| TEXAS INSTRUMENTS INCORPORATED
| Standard Linear and Logic Group
| IBIS Model of SN74AHC04
| HEX INVERTERS
| This file contains package information for the following:
|  SOIC 14-pin (D) package as [Component] AHC04_D
|  SSOP 14-pin (DB) package as [Component] AHC04_DB
|  TVSOP 14-pin (DGV) package as [Component] AHC04_DGV
|  PDIP 14-pin (N) package as [Component] AHC04_N
|  SOP 14-pin (NS) package as [Component] AHC04_NS
|  TSSOP 14-pin (PW) package as [Component] AHC04_PW
|  QFN 14-pin (RGY) package as [Component] AHC04_RGY
| This device can be powered at the following Vccs:
|  3.3 volt Vcc
|  5 volt Vcc
| This file provides unique models under the [Model Selector] for each Vcc.
| For operation at a specific Vcc, select the appropriate model after each
| [Model Selector] keyword.
[IBIS Ver]   3.2
[Comment char]  |_char
[File Name]   sn74ahc04.ibs
[File Rev]   1.1 | b_die
[Date]   May 16, 2003
[Source]   Data created from TI-SPICE simulations at TI-SLL.
[Notes]   The following is an IBIS list for the AHC04.
   Please contact sllibis@ti.com with questions and
   comments concerning SLL IBIS models.
   This IBIS model is created from a BA (back annotated
   netlist).
   - Power-clamp data has been deleted from the input model
[Disclaimer] Property of Texas Instruments Incorporated.  Unauthorized
   reproduction and/or distribution is strictly prohibited.
   This product is protected under copyright law.
   Created  2003, (C) Copyright  2003, Texas Instruments
   Incorporated, All Rights Reserved
   UNLESS THERE IS A SIGNED, WRITTEN AGREEMENT TO THE
   CONTRARY, TEXAS INSTRUMENTS (TI) IS PROVIDING THE IBIS
   MODELS  AND WITHOUT ANY WARRANTY, EXPRESSED OR
   IMPLIED.  TI assumes no liability for:
   1) the accuracy of the IBIS models provided to your
   company;
   2) the proper functioning of these IBIS Models in your
   design or for any resulting applications; or
   3) infringement of patents, copyrights or intellectual
   property rights resulting from your use of these IBIS
   models.
   TI provides IBIS Models as a service to our customers.
   You and your company shall not distribute, sell or give
   these models to anyone else without prior written
   permission from TI.
   TI reserves the right to make changes to our products or
   to discontinue any semiconductor product or service
   without notice, and advises our customers to obtain the
   latest version of relevant information to verify, before
   placing orders, that the information being relied on is
   current.
   Please be aware that your receipt and use of the IBIS
   information provided shall serve as acceptance of these
   terms and conditions.  If you do not accept these terms,
   you should return or destroy the IBIS models and any
   other accompanying information immediately.
| Component AHC04_D 14-pin SOIC
[Component]   AHC04_D
[Manufacturer]   Texas Instruments, Inc.
[Package]
|   typ   min   max
R_pkg   3.100e-02   2.800e-02   3.400e-02
L_pkg   3.109e-09   2.462e-09   3.889e-09
C_pkg   4.730e-13   3.630e-13   6.280e-13
[Pin]   signal_name   model_name   R_pin   L_pin   C_pin
1   1A   AHC04_IN   3.300e-02   3.854e-09   6.220e-13
2   1Y   AHC04_OUT   3.200e-02   3.188e-09   4.730e-13
3   2A   AHC04_IN   2.800e-02   2.462e-09   3.770e-13
4   2Y   AHC04_OUT   3.100e-02   2.596e-09   3.630e-13
5   3A   AHC04_IN   2.800e-02   2.521e-09   3.720e-13
6   3Y   AHC04_OUT   3.400e-02   3.250e-09   4.760e-13
7   GND   GND   3.400e-02   3.889e-09   6.280e-13
8   4Y   AHC04_OUT   3.400e-02   3.889e-09   6.280e-13
9   4A   AHC04_IN   3.400e-02   3.250e-09   4.760e-13
10   5Y   AHC04_OUT   2.800e-02   2.521e-09   3.720e-13
11   5A   AHC04_IN   3.100e-02   2.596e-09   3.640e-13
12   6Y   AHC04_OUT   2.800e-02   2.462e-09   3.770e-13
13   6A   AHC04_IN   3.200e-02   3.188e-09   4.730e-13
14   VCC   POWER   3.300e-02   3.854e-09   6.220e-13
| Component AHC04_DB 14-pin SSOP
[Component]   AHC04_DB
[Manufacturer]   Texas Instruments, Inc.
[Package]
|   typ   min   max
R_pkg   4.400e-02   4.100e-02   4.600e-02
L_pkg   3.551e-09   3.258e-09   3.927e-09
C_pkg   4.020e-13   3.600e-13   4.210e-13
[Pin]   signal_name   model_name   R_pin   L_pin   C_pin
1   1A   AHC04_IN   4.600e-02   3.927e-09   4.080e-13
2   1Y   AHC04_OUT   4.400e-02   3.587e-09   4.210e-13
3   2A   AHC04_IN   4.100e-02   3.289e-09   3.980e-13
4   2Y   AHC04_OUT   4.200e-02   3.258e-09   3.600e-13
5   3A   AHC04_IN   4.100e-02   3.286e-09   4.030e-13
6   3Y   AHC04_OUT   4.400e-02   3.586e-09   4.210e-13
7   GND   GND   4.600e-02   3.927e-09   4.080e-13
8   4Y   AHC04_OUT   4.600e-02   3.927e-09   4.080e-13
9   4A   AHC04_IN   4.400e-02   3.586e-09   4.210e-13
10   5Y   AHC04_OUT   4.100e-02   3.286e-09   4.030e-13
11   5A   AHC04_IN   4.300e-02   3.258e-09   3.600e-13
12   6Y   AHC04_OUT   4.100e-02   3.289e-09   3.980e-13
13   6A   AHC04_IN   4.400e-02   3.587e-09   4.210e-13
14   VCC   POWER   4.600e-02   3.927e-09   4.080e-13
| Component AHC04_DGV 14-pin TVSOP
[Component]   AHC04_DGV
[Manufacturer]   Texas Instruments, Inc.
[Package]
|   typ   min   max
R_pkg   3.500e-02   2.000e-02   4.500e-02
L_pkg   2.499e-09   2.077e-09   2.966e-09
C_pkg   3.610e-13   3.050e-13   4.160e-13
[Pin]   signal_name   model_name   R_pin   L_pin   C_pin
1   1A   AHC04_IN   2.700e-02   2.717e-09   3.730e-13
2   1Y   AHC04_OUT   3.700e-02   2.434e-09   3.980e-13
3   2A   AHC04_IN   3.400e-02   2.200e-09   3.160e-13
4   2Y   AHC04_OUT   2.000e-02   2.077e-09   3.090e-13
5   3A   AHC04_IN   3.000e-02   2.147e-09   3.050e-13
6   3Y   AHC04_OUT   4.200e-02   2.580e-09   4.080e-13
7   GND   GND   3.900e-02   2.921e-09   3.850e-13
8   4Y   AHC04_OUT   3.300e-02   2.841e-09   3.800e-13
9   4A   AHC04_IN   4.200e-02   2.611e-09   4.100e-13
10   5Y   AHC04_OUT   3.800e-02   2.331e-09   3.290e-13
11   5A   AHC04_IN   2.600e-02   2.223e-09   3.190e-13
12   6Y   AHC04_OUT   3.400e-02   2.259e-09   3.130e-13
13   6A   AHC04_IN   4.500e-02   2.681e-09   4.160e-13
14   VCC   POWER   4.200e-02   2.966e-09   3.860e-13
| Component AHC04_N 14-pin PDIP
[Component]   AHC04_N
[Manufacturer]   Texas Instruments, Inc.
[Package]
|   typ   min   max
R_pkg   4.500e-02   3.700e-02   6.300e-02
L_pkg   5.407e-09   3.922e-09   6.942e-09
C_pkg   3.890e-13   2.050e-13   6.040e-13
[Pin]   signal_name   model_name   R_pin   L_pin   C_pin
1   1A   AHC04_IN   6.300e-02   6.942e-09   6.040e-13
2   1Y   AHC04_OUT   3.700e-02   6.200e-09   4.060e-13
3   2A   AHC04_IN   4.200e-02   4.389e-09   3.220e-13
4   2Y   AHC04_OUT   3.800e-02   3.922e-09   2.050e-13
5   3A   AHC04_IN   3.900e-02   4.301e-09   2.980e-13
6   3Y   AHC04_OUT   3.800e-02   5.329e-09   3.560e-13
7   GND   GND   5.300e-02   6.510e-09   5.440e-13
8   4Y   AHC04_OUT   5.300e-02   6.437e-09   5.390e-13
9   4A   AHC04_IN   3.900e-02   5.352e-09   3.470e-13
10   5Y   AHC04_OUT   4.200e-02   4.473e-09   2.970e-13
11   5A   AHC04_IN   4.400e-02   4.326e-09   2.250e-13
12   6Y   AHC04_OUT   4.200e-02   4.295e-09   2.800e-13
13   6A   AHC04_IN   4.200e-02   6.318e-09   4.180e-13
14   VCC   POWER   6.100e-02   6.900e-09   6.030e-13
| Component AHC04_NS 14-pin SOP
[Component]   AHC04_NS
[Manufacturer]   Texas Instruments, Inc.
[Package]
|   typ   min   max
R_pkg   4.500e-02   3.900e-02   5.400e-02
L_pkg   3.796e-09   2.561e-09   4.952e-09
C_pkg   5.280e-13   2.880e-13   7.100e-13
[Pin]   signal_name   model_name   R_pin   L_pin   C_pin
1   1A   AHC04_IN   4.700e-02   4.867e-09   7.060e-13
2   1Y   AHC04_OUT   5.100e-02   4.083e-09   5.920e-13
3   2A   AHC04_IN   4.100e-02   2.915e-09   3.760e-13
4   2Y   AHC04_OUT   3.900e-02   2.561e-09   2.880e-13
5   3A   AHC04_IN   4.100e-02   3.101e-09   4.300e-13
6   3Y   AHC04_OUT   4.700e-02   4.047e-09   5.890e-13
7   GND   GND   5.100e-02   4.909e-09   7.000e-13
8   4Y   AHC04_OUT   4.500e-02   4.784e-09   6.940e-13
9   4A   AHC04_IN   5.400e-02   4.176e-09   5.970e-13
10   5Y   AHC04_OUT   3.900e-02   3.287e-09   4.490e-13
11   5A   AHC04_IN   3.900e-02   2.586e-09   2.940e-13
12   6Y   AHC04_OUT   4.000e-02   2.802e-09   3.710e-13
13   6A   AHC04_IN   4.900e-02   4.080e-09   5.930e-13
14   VCC   POWER   5.200e-02   4.952e-09   7.100e-13
| Component AHC04_PW 14-pin TSSOP
[Component]   AHC04_PW
[Manufacturer]   Texas Instruments, Inc.
[Package]
|   typ   min   max
R_pkg   3.200e-02   2.900e-02   3.500e-02
L_pkg   2.378e-09   2.170e-09   2.680e-09
C_pkg   3.140e-13   2.700e-13   3.350e-13
[Pin]   signal_name   model_name   R_pin   L_pin   C_pin
1   1A   AHC04_IN   3.300e-02   2.618e-09   3.300e-13
2   1Y   AHC04_OUT   3.100e-02   2.313e-09   3.170e-13
3   2A   AHC04_IN   3.000e-02   2.310e-09   3.140e-13
4   2Y   AHC04_OUT   3.100e-02   2.173e-09   2.720e-13
5   3A   AHC04_IN   3.000e-02   2.204e-09   3.090e-13
6   3Y   AHC04_OUT   3.200e-02   2.315e-09   3.170e-13
7   GND   GND   3.500e-02   2.680e-09   3.350e-13
8   4Y   AHC04_OUT   3.300e-02   2.640e-09   3.330e-13
9   4A   AHC04_IN   3.400e-02   2.347e-09   3.190e-13
10   5Y   AHC04_OUT   2.900e-02   2.277e-09   3.130e-13
11   5A   AHC04_IN   3.100e-02   2.170e-09   2.700e-13
12   6Y   AHC04_OUT   3.100e-02   2.244e-09   3.110e-13
13   6A   AHC04_IN   3.300e-02   2.343e-09   3.210e-13
14   VCC   POWER   3.500e-02   2.657e-09   3.320e-13
| Component AHC04_RGY 14-pin QFN
[Component]   AHC04_RGY
[Manufacturer]   Texas Instruments, Inc.
[Package]
|   typ   min   max
R_pkg   2.900e-02   2.300e-02   4.100e-02
L_pkg   7.730e-10   6.570e-10   9.980e-10
C_pkg   1.360e-13   1.150e-13   1.560e-13
[Pin]   signal_name   model_name   R_pin   L_pin   C_pin
1   1A   AHC04_IN   2.700e-02   8.310e-10   1.300e-13
2   1Y   AHC04_OUT   2.700e-02   8.660e-10   1.350e-13
3   2A   AHC04_IN   4.100e-02   9.980e-10   1.560e-13
4   2Y   AHC04_OUT   3.100e-02   7.670e-10   1.420e-13
5   3A   AHC04_IN   3.100e-02   7.650e-10   1.420e-13
6   3Y   AHC04_OUT   3.100e-02   7.830e-10   1.440e-13
7   GND   GND   3.100e-02   7.810e-10   1.370e-13
8   4Y   AHC04_OUT   2.300e-02   6.570e-10   1.150e-13
9   4A   AHC04_IN   2.300e-02   8.140e-10   1.290e-13
10   5Y   AHC04_OUT   2.800e-02   7.040e-10   1.290e-13
11   5A   AHC04_IN   2.700e-02   6.720e-10   1.360e-13
12   6Y   AHC04_OUT   2.700e-02   6.960e-10   1.380e-13
13   6A   AHC04_IN   2.700e-02   7.250e-10   1.400e-13
14   VCC   POWER   3.000e-02   7.630e-10   1.360e-13
| Model AHC04_IN
[Model Selector]   AHC04_IN
AHC04_IN_33   3.3 volt Vcc
AHC04_IN_50   5 volt Vcc
| Model AHC04_OUT
[Model Selector]   AHC04_OUT
AHC04_OUT_33   3.3 volt Vcc
AHC04_OUT_50   5 volt Vcc
| Models and submodels in the file (4): AHC04_IN_33 (Input), AHC04_IN_50 (Input), AHC04_OUT_33 (Output), AHC04_OUT_50 (Output)
